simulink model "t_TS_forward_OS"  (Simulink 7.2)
settings: Solver=ode3  SolverMode=SingleTasking  StartTime=0.0  StopTime=0.01  FixedStep=10e-6  MaxStep=5e-6  RelTol=1e-6  AbsTol=1e-6

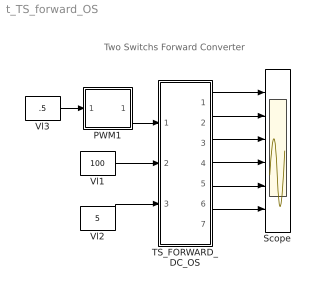
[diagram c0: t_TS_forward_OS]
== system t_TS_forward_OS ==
  note: Two Switchs Forward Converter
  PWM1 : Subsystem  mask(PWMtr){FS=2.5e3}
      mask prompts: FS "Frequency"
  Scope : Scope  NumInputPorts=6
  TS_FORWARD_DC_OS : Subsystem  mask{L1=2e-3, L2=4*2e-3, KP=1, L=5e-3, iL0=20, C=2e-4, UC0=100, R=5}
      mask prompts: L1 "Inductance L1"; L2 "Inductance L2"; KP "Coupling Coeff KP"; L "Inductance"; iL0 "Initial Ind. Current"; C "Cap"; UC0 "initial Cap Voltage"; R "Load Resistance"
      mask help: Two Switchs Forward Converter Input Vector u: u[0]= T1.gate and T2.gate u[1]= E.v u[2]= IDC.i Output Vector y: y[0]= T1.I y[1]= D1.I y[2]= T2.I y[3]= D2.I y[4]= L1.I y[5]= C1.V y[6]= E.I Parameter Vector p: p[0]= Mut_L1.L1 p[1]= Mut_L2.L2 p[2]= Mut_Coupling Coeff.k p[3]= L1.L p[4]= L1.iL10 p[5]= C1.C p[6]= C1.vC0 p[7]= R1.r You can pause the simulation during running, change the Parameters you want and continue the Simulation
  Vl1 : Constant  Value=100
  Vl2 : Constant  Value=5
  Vl3 : Constant  Value=.5
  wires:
  Vl3/1 -> PWM1/1(In1)
  PWM1/1(Out1) -> TS_FORWARD_DC_OS/1(sw)
  Vl1/1 -> TS_FORWARD_DC_OS/2(E)
  TS_FORWARD_DC_OS/1(iT1) -> Scope/1
  TS_FORWARD_DC_OS/2(iD1) -> Scope/2
  TS_FORWARD_DC_OS/3(iT2) -> Scope/3
  TS_FORWARD_DC_OS/4(iD2) -> Scope/4
  TS_FORWARD_DC_OS/5(iL1) -> Scope/5
  TS_FORWARD_DC_OS/6(vC) -> Scope/6
  Vl2/1 -> TS_FORWARD_DC_OS/3(IDC)

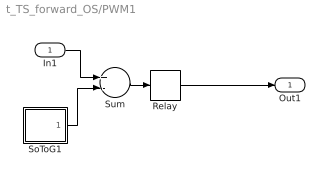
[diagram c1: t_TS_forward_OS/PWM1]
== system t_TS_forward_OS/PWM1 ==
  In1 : Inport
  Relay : Relay
  SoToG1 : Subsystem  mask(SoToG){T=1e-3}
      mask prompts: T "Period Time"
  Sum : Sum  Inputs=+-
  Out1 : Outport  InitialOutput=0
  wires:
  Relay/1 -> Out1/1
  SoToG1/1(O) -> Sum/2
  In1/1 -> Sum/1
  Sum/1 -> Relay/1

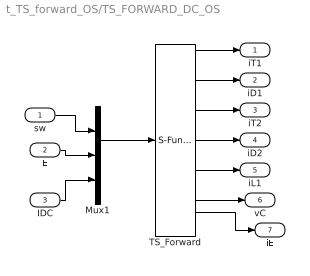
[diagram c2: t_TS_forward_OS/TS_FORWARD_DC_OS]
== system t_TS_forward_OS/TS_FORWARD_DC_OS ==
  sw : Inport  OutDataType=sfix(16)  OutScaling=2^0
  E : Inport  Port=2  OutDataType=sfix(16)  OutScaling=2^0
  IDC : Inport  Port=3  OutDataType=sfix(16)  OutScaling=2^0
  Mux1 : Mux  Inputs=3
  TS_Forward : S-Function  FunctionName=s_TS_forward_OS  Parameters="[L1  L2   KP  L iL0  C  UC0  R]"  EnableBusSupport=off
  iT1 : Outport  OutDataType=sfix(16)  OutScaling=2^0
  iD1 : Outport  Port=2  OutDataType=sfix(16)  OutScaling=2^0
  iT2 : Outport  Port=3  OutDataType=sfix(16)  OutScaling=2^0
  iD2 : Outport  Port=4  OutDataType=sfix(16)  OutScaling=2^0
  iL1 : Outport  Port=5  OutDataType=sfix(16)  OutScaling=2^0
  vC : Outport  Port=6  OutDataType=sfix(16)  OutScaling=2^0
  iE : Outport  Port=7  OutDataType=sfix(16)  OutScaling=2^0
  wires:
  sw/1 -> Mux1/1
  Mux1/1 -> TS_Forward/1
  E/1 -> Mux1/2
  TS_Forward/1 -> iT1/1
  TS_Forward/2 -> iD1/1
  TS_Forward/3 -> iT2/1
  TS_Forward/4 -> iD2/1
  TS_Forward/5 -> iL1/1
  TS_Forward/6 -> vC/1
  IDC/1 -> Mux1/3
  TS_Forward/7 -> iE/1

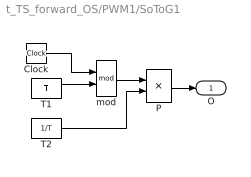
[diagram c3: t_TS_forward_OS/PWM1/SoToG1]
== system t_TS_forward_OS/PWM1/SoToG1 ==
  Clock : Clock
  P : Product
  T1 : Constant  Value=T
  T2 : Constant  Value=1/T
  mod : Math  Operator=mod
  O : Outport
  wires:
  Clock/1 -> mod/1
  T1/1 -> mod/2
  T2/1 -> P/2
  mod/1 -> P/1
  P/1 -> O/1
